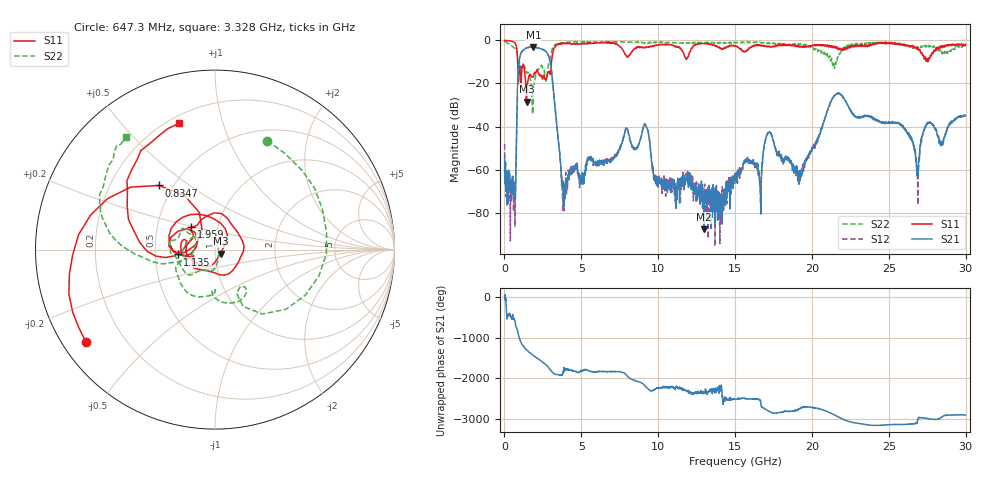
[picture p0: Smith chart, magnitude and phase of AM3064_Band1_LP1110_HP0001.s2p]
# Hz S DB R 50.0
!freq dBS11 angS11 dBS21 angS21 dBS12 angS12 dBS22 angS22
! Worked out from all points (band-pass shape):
!   1600 points, 10 MHz to 29.98 GHz, reference 50 ohm
!   highest |S21| = -3.05 dB at 1.884 GHz (marker M1); lowest = -87.6 dB at 12.96 GHz (marker M2)
!   |S21| within 3 dB of the highest: 1.066 GHz to 2.79 GHz (1.724 GHz wide, 89.4 % of centre)
!   lowest |S11| = -28.5 dB at 1.435 GHz (marker M3), VSWR 1.08, Z = 53.1 - j2.33 ohm
!   |S11| at or under -10 dB: 857.5 MHz to 3.06 GHz (2.203 GHz wide, 112 % of centre)
!   |S22| runs from -34.2 to -0.4 dB; largest |S21 - S12| = 0.011
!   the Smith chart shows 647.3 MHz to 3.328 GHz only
!   S11 on the Smith chart (normalised r, x): 647.3 MHz: 0.07, -0.32; 834.7 MHz: 0.42, +0.39; 1.135 GHz: 0.66, -0.04; 1.959 GHz: 0.75, +0.19; 3.328 GHz: 0.24, +0.73
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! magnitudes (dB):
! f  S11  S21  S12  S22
! 10 MHz  -0.1  -53.7  -48.1  -0.4
! 647.3 MHz  -1.1  -65.8  -68.1  -3.4
! 834.7 MHz  -6.5  -27.7  -27.6  -7.0
! 1.135 GHz  -13.6  -5.2  -5.2  -12.2
! 1.435 GHz  -28.5  -3.5  -3.4  -15.2
! 1.884 GHz  -16.8  -3.1  -3.2  -25.9
! 1.959 GHz  -14.9  -3.2  -3.2  -18.8
! 2.878 GHz  -14.4  -7.3  -7.3  -10.5
! 3.328 GHz  -2.7  -33.9  -34.0  -2.0
! 3.834 GHz  -1.4  -76.3  -65.4  -1.1
! 5.015 GHz  -1.6  -64.8  -65.3  -0.7
! 9.157 GHz  -3.4  -38.9  -39.0  -1.1
! 10 GHz  -2.2  -68.0  -64.8  -0.9
! 12.96 GHz  -1.5  -87.6  -74.8  -1.0
! 15 GHz  -2.6  -62.7  -63.5  -1.2
! 16.64 GHz  -2.4  -69.0  -67.7  -0.9
! 17.2 GHz  -2.6  -42.7  -42.6  -1.1
! 19.99 GHz  -2.7  -50.8  -51.7  -3.1
! 21.64 GHz  -3.3  -24.8  -24.8  -8.6
! 25 GHz  -1.0  -38.2  -37.6  -1.0
! 26.87 GHz  -4.1  -61.7  -64.6  -3.0
! 29.98 GHz  -1.8  -35.0  -35.0  -2.9
